FUNCTION "CENTR. 2  ANTERIORE SX" : VOID
TITLE =
VERSION : 0.1

BEGIN
NETWORK
TITLE =LETTURA STATUS WORD DA DRIVE
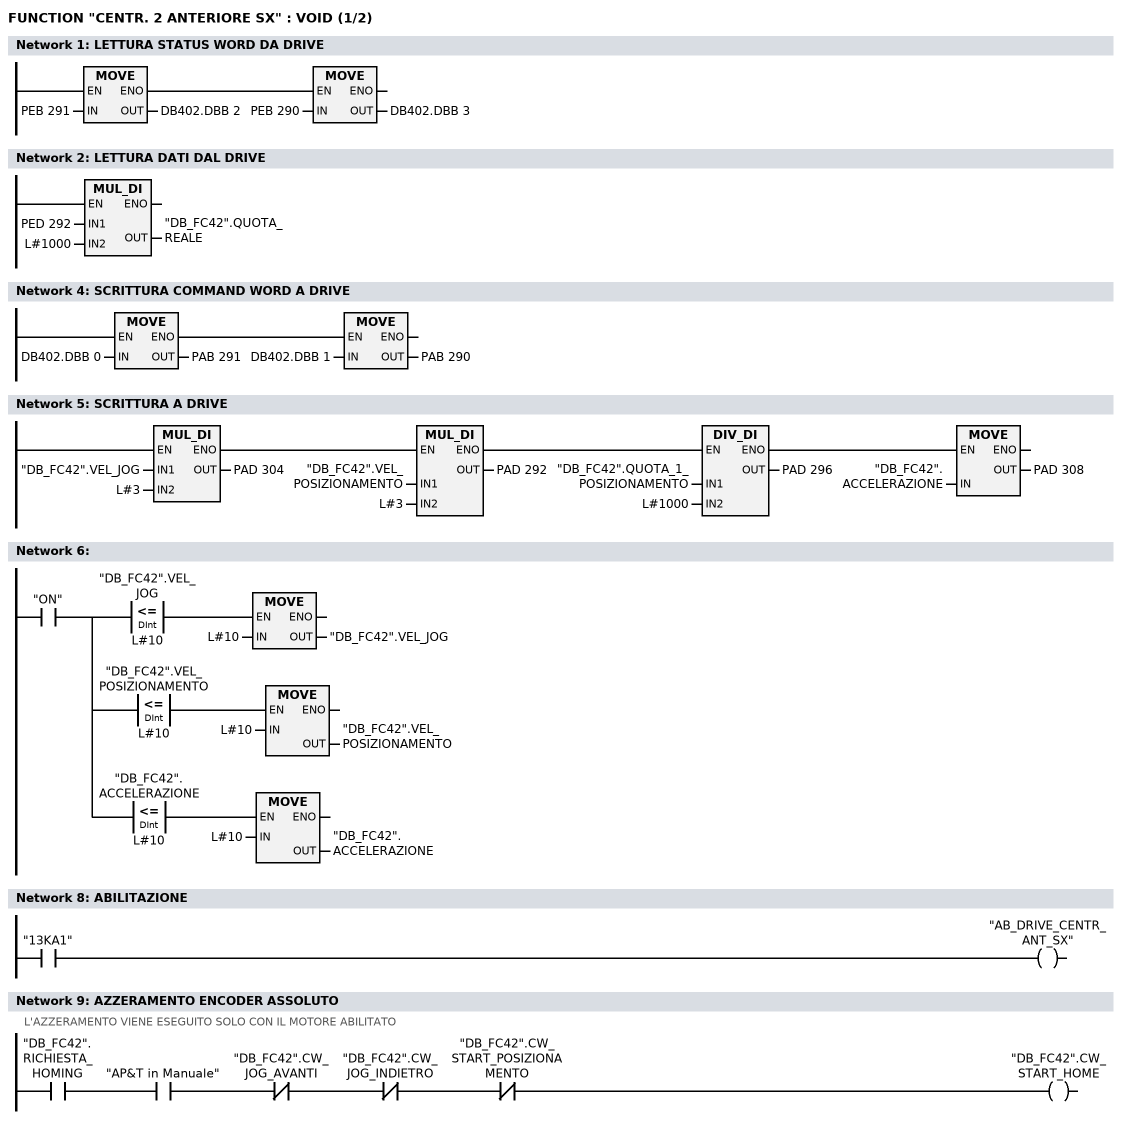
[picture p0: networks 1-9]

      U(    ;
      L     PEB  291;
      T     DB402.DBB    2;
      SET   ;
      SAVE  ;
      CLR   ;
      U     BIE;
      )     ;
      SPBNB _001;
      L     PEB  290;
      T     DB402.DBB    3;
_001: NOP   0;
NETWORK
TITLE =LETTURA DATI DAL DRIVE

      L     PED  292;
      L     L#1000;
      *D    ;
      T     "DB_FC42".QUOTA_REALE;
      NOP   0;
NETWORK
TITLE =

NETWORK
TITLE =SCRITTURA COMMAND WORD A DRIVE

      U(    ;
      L     DB402.DBB    0;
      T     PAB  291;
      SET   ;
      SAVE  ;
      CLR   ;
      U     BIE;
      )     ;
      SPBNB _002;
      L     DB402.DBB    1;
      T     PAB  290;
_002: NOP   0;
NETWORK
TITLE =SCRITTURA A DRIVE

      U(    ;
      U(    ;
      U(    ;
      L     "DB_FC42".VEL_JOG;
      L     L#3;
      *D    ;
      T     PAD  304;
      UN    OV;
      SAVE  ;
      CLR   ;
      U     BIE;
      )     ;
      SPBNB _003;
      L     "DB_FC42".VEL_POSIZIONAMENTO;
      L     L#3;
      *D    ;
      T     PAD  292;
      UN    OV;
      SAVE  ;
      CLR   ;
_003: U     BIE;
      )     ;
      SPBNB _004;
      L     "DB_FC42".QUOTA_1_POSIZIONAMENTO;
      L     L#1000;
      /D    ;
      T     PAD  296;
      UN    OV;
      SAVE  ;
      CLR   ;
_004: U     BIE;
      )     ;
      SPBNB _005;
      L     "DB_FC42".ACCELERAZIONE;
      T     PAD  308;
_005: NOP   0;
NETWORK
TITLE =

      U     "ON";
      =     L      0.0;
      U     L      0.0;
      U(    ;
      L     "DB_FC42".VEL_JOG;
      L     L#10;
      <=D   ;
      )     ;
      SPBNB _006;
      L     L#10;
      T     "DB_FC42".VEL_JOG;
_006: NOP   0;
      U     L      0.0;
      U(    ;
      L     "DB_FC42".VEL_POSIZIONAMENTO;
      L     L#10;
      <=D   ;
      )     ;
      SPBNB _007;
      L     L#10;
      T     "DB_FC42".VEL_POSIZIONAMENTO;
_007: NOP   0;
      U     L      0.0;
      U(    ;
      L     "DB_FC42".ACCELERAZIONE;
      L     L#10;
      <=D   ;
      )     ;
      SPBNB _008;
      L     L#10;
      T     "DB_FC42".ACCELERAZIONE;
_008: NOP   0;
NETWORK
TITLE =

NETWORK
TITLE =ABILITAZIONE

      U     "13KA1";
      =     "AB_DRIVE_CENTR_ANT_SX";
NETWORK
TITLE =AZZERAMENTO ENCODER ASSOLUTO
//L'AZZERAMENTO VIENE ESEGUITO SOLO CON IL MOTORE ABILITATO
      U     "DB_FC42".RICHIESTA_HOMING;
      U     "AP&T in Manuale";
      UN    "DB_FC42".CW_JOG_AVANTI;
      UN    "DB_FC42".CW_JOG_INDIETRO;
      UN    "DB_FC42".CW_START_POSIZIONAMENTO;
      =     "DB_FC42".CW_START_HOME;
NETWORK
TITLE =COMANDI DI JOG
//N.B. VERIFICARE QUOTE EXTRACORSA SOFTWARE
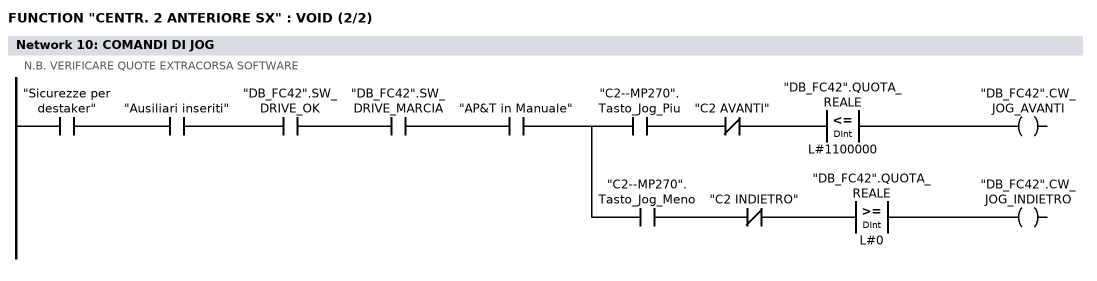
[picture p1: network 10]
      U     "Sicurezze per destaker";
      U     "Ausiliari inseriti";
      U     "DB_FC42".SW_DRIVE_OK;
      U     "DB_FC42".SW_DRIVE_MARCIA;
      U     "AP&T in Manuale";
      =     L      0.0;
      U     L      0.0;
      U     "C2--MP270".Tasto_Jog_Piu;
      UN    "C2 AVANTI";
      U(    ;
      L     "DB_FC42".QUOTA_REALE;
      L     L#1100000;
      <=D   ;
      )     ;
      =     "DB_FC42".CW_JOG_AVANTI;
      U     L      0.0;
      U     "C2--MP270".Tasto_Jog_Meno;
      UN    "C2 INDIETRO";
      U(    ;
      L     "DB_FC42".QUOTA_REALE;
      L     L#0;
      >=D   ;
      )     ;
      =     "DB_FC42".CW_JOG_INDIETRO;
NETWORK
TITLE =Centratore 2: Posizioni

      U     "ON";
      =     L      0.0;
      U     L      0.0;
      U(    ;
      L     "DB_FC42".QUOTA_REALE;
      L     L#100;
      <=D   ;
      )     ;
      U(    ;
      L     "DB_FC42".QUOTA_REALE;
      L     L#-100;
      >=D   ;
      )     ;
      =     "C2: Asse in pos.0";
      U(    ;
      U(    ;
      U     L      0.0;
      SPBNB _009;
      L     "MATRICOLA ATTUALE".C2_Posizione_1;
      L     L#100;
      -D    ;
      T     "CONFRONTI CENTRATORI".C2_Pos_1_Min;
      UN    OV;
      SAVE  ;
      CLR   ;
_009: U     BIE;
      )     ;
      SPBNB _00a;
      L     "MATRICOLA ATTUALE".C2_Posizione_1;
      L     L#200;
      +D    ;
      T     "CONFRONTI CENTRATORI".C2_Pos_1_Max;
      UN    OV;
      SAVE  ;
      CLR   ;
_00a: U     BIE;
      )     ;
      U(    ;
      L     "DB_FC42".QUOTA_REALE;
      L     "CONFRONTI CENTRATORI".C2_Pos_1_Min;
      >=D   ;
      )     ;
      U(    ;
      L     "DB_FC42".QUOTA_REALE;
      L     "CONFRONTI CENTRATORI".C2_Pos_1_Max;
      <=D   ;
      )     ;
      =     "C2: Asse in pos.1";
      U(    ;
      U(    ;
      U     L      0.0;
      SPBNB _00b;
      L     "MATRICOLA ATTUALE".C2_Posizione_2;
      L     L#100;
      -D    ;
      T     "CONFRONTI CENTRATORI".C2_Pos_2_Min;
      UN    OV;
      SAVE  ;
      CLR   ;
_00b: U     BIE;
      )     ;
      SPBNB _00c;
      L     "MATRICOLA ATTUALE".C2_Posizione_2;
      L     L#50000;
      +D    ;
      T     "CONFRONTI CENTRATORI".C2_Pos_2_Max;
      UN    OV;
      SAVE  ;
      CLR   ;
_00c: U     BIE;
      )     ;
      U(    ;
      L     "DB_FC42".QUOTA_REALE;
      L     "CONFRONTI CENTRATORI".C2_Pos_2_Min;
      >=D   ;
      )     ;
      UN    "C2: Asse in pos.3";
      UN    "C2: Asse in pos.4";
      =     "C2: Asse in pos.2";
      U(    ;
      U(    ;
      U     L      0.0;
      SPBNB _00d;
      L     "MATRICOLA ATTUALE".C2_Posizione_3;
      L     L#100;
      -D    ;
      T     "CONFRONTI CENTRATORI".C2_Pos_3_Min;
      UN    OV;
      SAVE  ;
      CLR   ;
_00d: U     BIE;
      )     ;
      SPBNB _00e;
      L     "MATRICOLA ATTUALE".C2_Posizione_3;
      L     L#50000;
      +D    ;
      T     "CONFRONTI CENTRATORI".C2_Pos_3_Max;
      UN    OV;
      SAVE  ;
      CLR   ;
_00e: U     BIE;
      )     ;
      U(    ;
      L     "DB_FC42".QUOTA_REALE;
      L     "CONFRONTI CENTRATORI".C2_Pos_3_Min;
      >=D   ;
      )     ;
      UN    "C2: Asse in pos.4";
      =     "C2: Asse in pos.3";
      U(    ;
      U(    ;
      U     L      0.0;
      SPBNB _00f;
      L     "MATRICOLA ATTUALE".C2_Posizione_4;
      L     L#100;
      -D    ;
      T     "CONFRONTI CENTRATORI".C2_Pos_4_Min;
      UN    OV;
      SAVE  ;
      CLR   ;
_00f: U     BIE;
      )     ;
      SPBNB _010;
      L     "MATRICOLA ATTUALE".C2_Posizione_4;
      L     L#100;
      +D    ;
      T     "CONFRONTI CENTRATORI".C2_Pos_4_Max;
      UN    OV;
      SAVE  ;
      CLR   ;
_010: U     BIE;
      )     ;
      U(    ;
      L     "DB_FC42".QUOTA_REALE;
      L     "CONFRONTI CENTRATORI".C2_Pos_4_Min;
      >=D   ;
      )     ;
      U(    ;
      L     "DB_FC42".QUOTA_REALE;
      L     "CONFRONTI CENTRATORI".C2_Pos_4_Max;
      <=D   ;
      )     ;
      =     "C2: Asse in pos.4";
NETWORK
TITLE =Centratore 2: consenso abilitazione passi
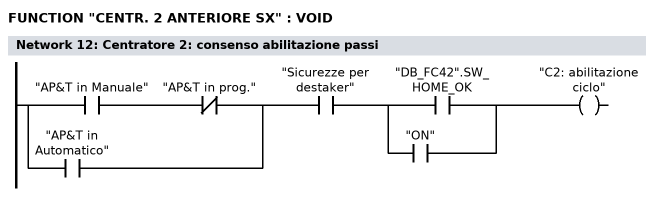
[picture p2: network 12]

      U(    ;
      U     "AP&T in Manuale";
      UN    "AP&T in prog.";
      O     "AP&T in Automatico";
      )     ;
      U     "Sicurezze per destaker";
      U(    ;
      O     "DB_FC42".SW_HOME_OK;
      O     "ON";
      )     ;
      =     "C2: abilitazione ciclo";
NETWORK
TITLE =Centratore 2: comando avvicinamento  (centraggi aperti)

      U(    ;
      U(    ;
      O     "Comando apre centraggi";
      O     "C2--MP270".Tasto_Indietro;
      O     ;
      U     "Apertura centratori";
      U(    ;
      O     "Centratori a riposo";
      O     "Centratori tutti chiusi";
      )     ;
      )     ;
      UN    "C2: Asse in pos.1";
      UN    "C2: comando arrivo";
      UN    "C2: comando a riposo";
      U     "C2: abilitazione ciclo";
      L     S5T#100MS;
      SE    T    183;
      NOP   0;
      NOP   0;
      NOP   0;
      U     T    183;
      )     ;
      S     "C2: comando avvicinam";
      U(    ;
      O     "C2: Asse in pos.1";
      O(    ;
      U(    ;
      O     "Ripristino centratori";
      O     "Comando riposo centraggi";
      O     "C2--MP270".Tasto_Riposo;
      )     ;
      FP    "C2: one shot 1";
      )     ;
      )     ;
      R     "C2: comando avvicinam";
      NOP   0;
NETWORK
TITLE =Centratore 2: comando arrivo (centraggi chiusi)

      U(    ;
      U(    ;
      O     "Comando chiude centraggi";
      O     "C2--MP270".Tasto_Avanti;
      O     ;
      U     "Chiusura centratori";
      U(    ;
      O     "Centratori tutti aperti";
      O     "Centratori a riposo";
      )     ;
      )     ;
      UN    "C2: Asse in pos.4";
      UN    "C2: comando avvicinam";
      UN    "C2: comando a riposo";
      U     "C2: abilitazione ciclo";
      L     S5T#100MS;
      SE    T    184;
      NOP   0;
      NOP   0;
      NOP   0;
      U     T    184;
      )     ;
      S     "C2: comando arrivo";
      U(    ;
      O     "C2: Asse in pos.4";
      O(    ;
      U(    ;
      O     "Ripristino centratori";
      O     "Comando riposo centraggi";
      O     "C2--MP270".Tasto_Riposo;
      )     ;
      FP    "C2: one shot 2";
      )     ;
      )     ;
      R     "C2: comando arrivo";
      NOP   0;
NETWORK
TITLE =Centratore 2: comando automatico centraggi a riposo

      U(    ;
      U(    ;
      O     "Comando riposo centraggi";
      O     "C2--MP270".Tasto_Riposo;
      )     ;
      UN    "C2: Asse in pos.0";
      UN    "C2: comando avvicinam";
      UN    "C2: comando arrivo";
      U     "C2: abilitazione ciclo";
      L     S5T#100MS;
      SE    T    185;
      NOP   0;
      NOP   0;
      NOP   0;
      U     T    185;
      )     ;
      S     "C2: comando a riposo";
      U(    ;
      O     "C2: Asse in pos.0";
      O(    ;
      U     "Ripristino centratori";
      FP    "C2: one shot 3";
      )     ;
      )     ;
      R     "C2: comando a riposo";
      NOP   0;
NETWORK
TITLE =Centratore 2: quote impostate per posizioni

      U     "ON";
      =     L      0.0;
      U(    ;
      U(    ;
      U     L      0.0;
      U     "C2: comando a riposo";
      UN    "C2: Asse in pos.0";
      SPBNB _011;
      L     0;
      T     "DB_FC42".QUOTA_1_POSIZIONAMENTO;
      SET   ;
      SAVE  ;
      CLR   ;
_011: U     BIE;
      )     ;
      SPBNB _012;
      L     L#150;
      T     "DB_FC42".VEL_POSIZIONAMENTO;
      SET   ;
      SAVE  ;
      CLR   ;
_012: U     BIE;
      )     ;
      SPBNB _013;
      L     L#1000;
      T     "DB_FC42".ACCELERAZIONE;
      SET   ;
      SAVE  ;
      CLR   ;
_013: U     BIE;
      =     "C2: Quote pronte pos.0";
      U(    ;
      U(    ;
      U     L      0.0;
      U     "C2: comando avvicinam";
      UN    "C2: Asse in pos.1";
      SPBNB _014;
      L     "MATRICOLA ATTUALE".C2_Posizione_1;
      T     "DB_FC42".QUOTA_1_POSIZIONAMENTO;
      SET   ;
      SAVE  ;
      CLR   ;
_014: U     BIE;
      )     ;
      SPBNB _015;
      L     "MATRICOLA ATTUALE".C2_Velocita_1;
      T     "DB_FC42".VEL_POSIZIONAMENTO;
      SET   ;
      SAVE  ;
      CLR   ;
_015: U     BIE;
      )     ;
      SPBNB _016;
      L     "MATRICOLA ATTUALE".C2_Accell_1;
      T     "DB_FC42".ACCELERAZIONE;
      SET   ;
      SAVE  ;
      CLR   ;
_016: U     BIE;
      =     "C2: Quote pronte pos.1";
      U     L      0.0;
      U     "C2: comando arrivo";
      =     L      0.1;
      U(    ;
      U(    ;
      U     L      0.1;
      UN    "C2: Asse in pos.2";
      SPBNB _017;
      L     "MATRICOLA ATTUALE".C2_Posizione_4;
      T     "DB_FC42".QUOTA_1_POSIZIONAMENTO;
      SET   ;
      SAVE  ;
      CLR   ;
_017: U     BIE;
      )     ;
      SPBNB _018;
      L     "MATRICOLA ATTUALE".C2_Velocita_2;
      T     "DB_FC42".VEL_POSIZIONAMENTO;
      SET   ;
      SAVE  ;
      CLR   ;
_018: U     BIE;
      )     ;
      SPBNB _019;
      L     "MATRICOLA ATTUALE".C2_Accell_2;
      T     "DB_FC42".ACCELERAZIONE;
      SET   ;
      SAVE  ;
      CLR   ;
_019: U     BIE;
      S     "C2: Quote pronte pos.2";
      U     L      0.1;
      U     "C2: Quote pronte pos.2";
      UN    "C2: Reset start pos.2";
      L     S5T#1S;
      SE    "C2: ritardo P2";
      NOP   0;
      NOP   0;
      NOP   0;
      U     "C2: ritardo P2";
      S     "C2: Reset start pos.2";
      R     "C2: Quote pronte pos.2";
      U     L      0.0;
      U     "C2: comando arrivo";
      =     L      0.1;
      U(    ;
      U(    ;
      U(    ;
      U     L      0.1;
      U     "C2: Asse in pos.2";
      UN    "C2: Asse in pos.3";
      SPBNB _01a;
      L     "MATRICOLA ATTUALE".C2_Posizione_4;
      T     "DB_FC42".QUOTA_1_POSIZIONAMENTO;
      SET   ;
      SAVE  ;
      CLR   ;
_01a: U     BIE;
      )     ;
      SPBNB _01b;
      L     "MATRICOLA ATTUALE".C2_Velocita_3;
      T     "DB_FC42".VEL_POSIZIONAMENTO;
      SET   ;
      SAVE  ;
      CLR   ;
_01b: U     BIE;
      )     ;
      SPBNB _01c;
      L     "MATRICOLA ATTUALE".C2_Accell_3;
      T     "DB_FC42".ACCELERAZIONE;
      SET   ;
      SAVE  ;
      CLR   ;
_01c: U     BIE;
      )     ;
      U     "C2: Reset start pos.2";
      S     "C2: Quote pronte pos.3";
      R     "C2: Reset start pos.2";
      U     L      0.1;
      U     "C2: Quote pronte pos.3";
      L     S5T#500MS;
      SE    "C2: ritardo P3";
      NOP   0;
      NOP   0;
      NOP   0;
      U     "C2: ritardo P3";
      S     "C2: Reset start pos.3";
      R     "C2: Quote pronte pos.3";
      U     L      0.0;
      U     "C2: comando arrivo";
      =     L      0.1;
      U(    ;
      U(    ;
      U(    ;
      U     L      0.1;
      U     "C2: Asse in pos.3";
      UN    "C2: Asse in pos.4";
      SPBNB _01d;
      L     "MATRICOLA ATTUALE".C2_Posizione_4;
      T     "DB_FC42".QUOTA_1_POSIZIONAMENTO;
      SET   ;
      SAVE  ;
      CLR   ;
_01d: U     BIE;
      )     ;
      SPBNB _01e;
      L     "MATRICOLA ATTUALE".C2_Velocita_4;
      T     "DB_FC42".VEL_POSIZIONAMENTO;
      SET   ;
      SAVE  ;
      CLR   ;
_01e: U     BIE;
      )     ;
      SPBNB _01f;
      L     "MATRICOLA ATTUALE".C2_Accell_4;
      T     "DB_FC42".ACCELERAZIONE;
      SET   ;
      SAVE  ;
      CLR   ;
_01f: U     BIE;
      )     ;
      U     "C2: Reset start pos.3";
      S     "C2: Quote pronte pos.4";
      R     "C2: Reset start pos.3";
      U     L      0.1;
      U     "C2: Quote pronte pos.4";
      L     S5T#500MS;
      SE    "C2: ritardo P4";
      NOP   0;
      NOP   0;
      NOP   0;
      U     "C2: ritardo P4";
      S     "C2: Reset start pos.4";
      R     "C2: Quote pronte pos.4";
NETWORK
TITLE =Centratore 2: reset impostate
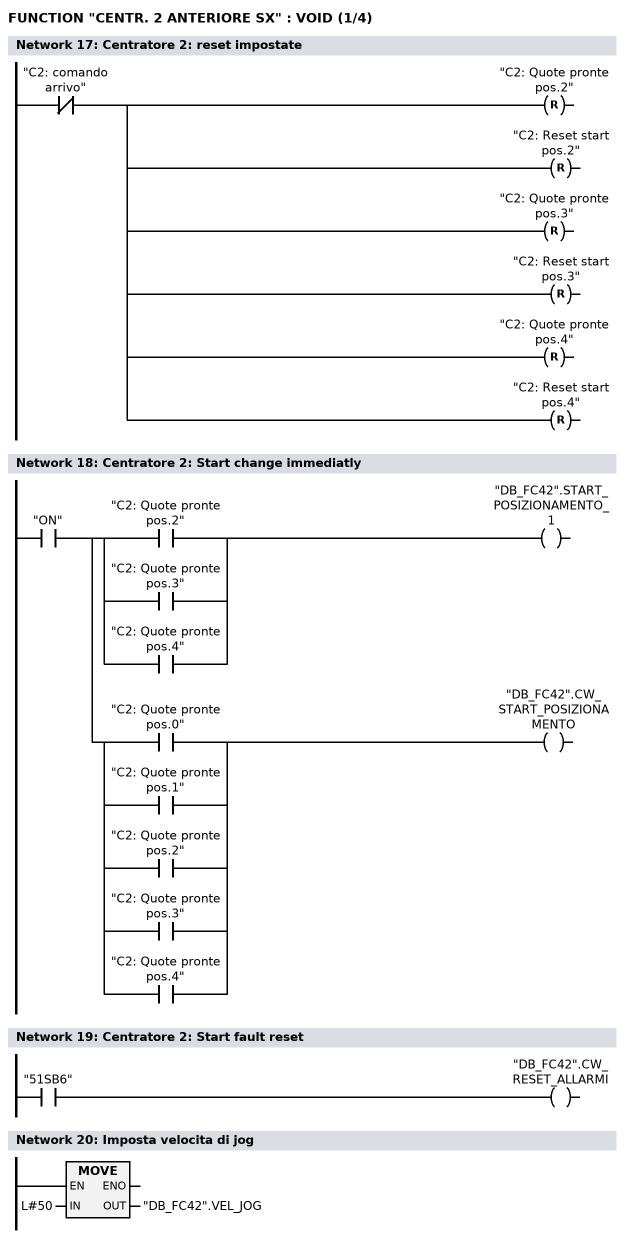
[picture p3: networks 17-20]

      UN    "C2: comando arrivo";
      R     "C2: Quote pronte pos.2";
      R     "C2: Reset start pos.2";
      R     "C2: Quote pronte pos.3";
      R     "C2: Reset start pos.3";
      R     "C2: Quote pronte pos.4";
      R     "C2: Reset start pos.4";
NETWORK
TITLE =Centratore 2: Start change immediatly

      U     "ON";
      =     L      0.0;
      U     L      0.0;
      U(    ;
      O     "C2: Quote pronte pos.2";
      O     "C2: Quote pronte pos.3";
      O     "C2: Quote pronte pos.4";
      )     ;
      =     "DB_FC42".START_POSIZIONAMENTO_1;
      U     L      0.0;
      U(    ;
      O     "C2: Quote pronte pos.0";
      O     "C2: Quote pronte pos.1";
      O     "C2: Quote pronte pos.2";
      O     "C2: Quote pronte pos.3";
      O     "C2: Quote pronte pos.4";
      )     ;
      =     "DB_FC42".CW_START_POSIZIONAMENTO;
NETWORK
TITLE =Centratore 2: Start fault reset

      U     "51SB6";
      =     "DB_FC42".CW_RESET_ALLARMI;
NETWORK
TITLE =Imposta velocita di jog

      L     L#50;
      T     "DB_FC42".VEL_JOG;
      NOP   0;
NETWORK
TITLE =Centratore 1: Drive Enable ok
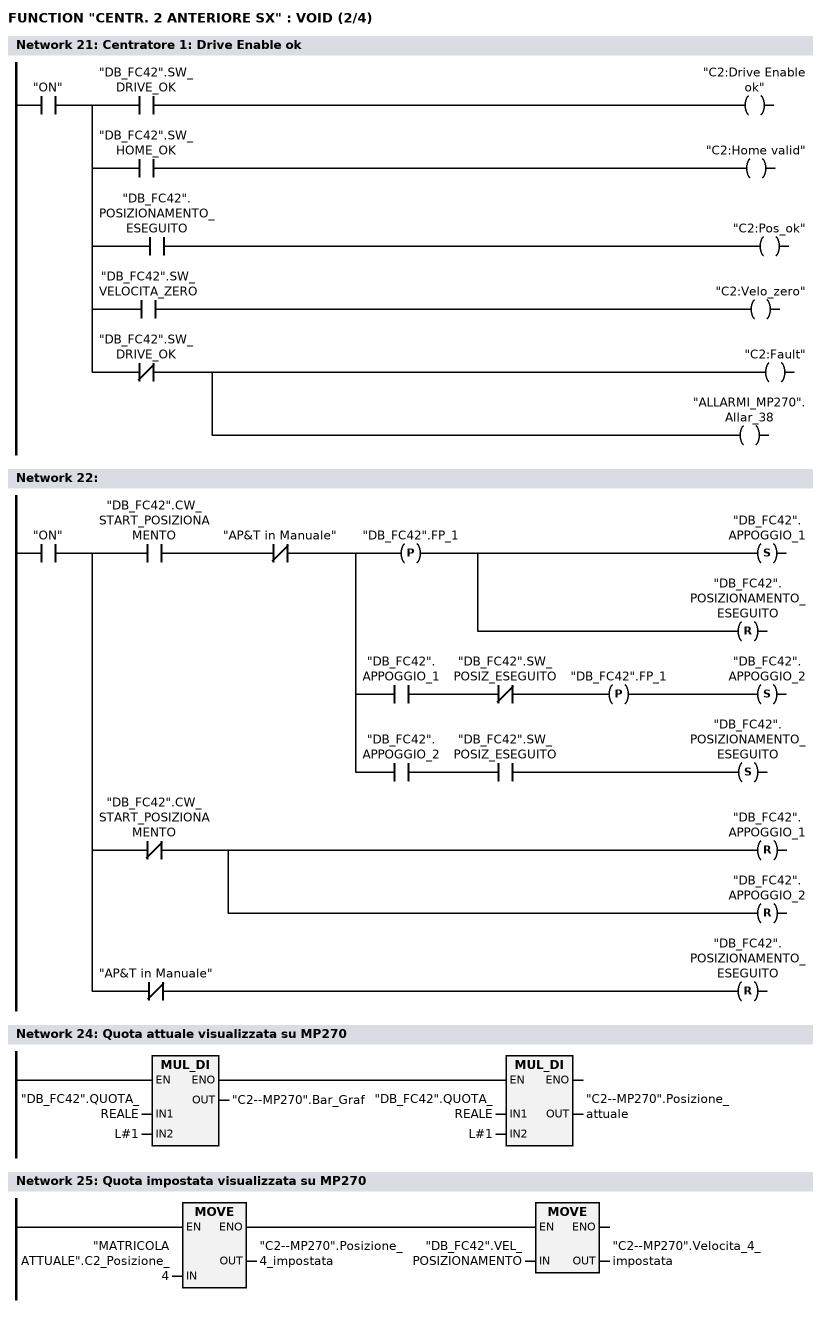
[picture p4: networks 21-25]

      U     "ON";
      =     L      0.0;
      U     L      0.0;
      U     "DB_FC42".SW_DRIVE_OK;
      =     "C2:Drive Enable ok";
      U     L      0.0;
      U     "DB_FC42".SW_HOME_OK;
      =     "C2:Home valid";
      U     L      0.0;
      U     "DB_FC42".POSIZIONAMENTO_ESEGUITO;
      =     "C2:Pos_ok";
      U     L      0.0;
      U     "DB_FC42".SW_VELOCITA_ZERO;
      =     "C2:Velo_zero";
      U     L      0.0;
      UN    "DB_FC42".SW_DRIVE_OK;
      =     "C2:Fault";
      =     "ALLARMI_MP270".Allar_38;
NETWORK
TITLE =

      U     "ON";
      =     L      0.0;
      U     L      0.0;
      U     "DB_FC42".CW_START_POSIZIONAMENTO;
      UN    "AP&T in Manuale";
      =     L      0.1;
      U     L      0.1;
      FP    "DB_FC42".FP_1;
      S     "DB_FC42".APPOGGIO_1;
      R     "DB_FC42".POSIZIONAMENTO_ESEGUITO;
      U     L      0.1;
      U     "DB_FC42".APPOGGIO_1;
      UN    "DB_FC42".SW_POSIZ_ESEGUITO;
      FP    "DB_FC42".FP_1;
      S     "DB_FC42".APPOGGIO_2;
      U     L      0.1;
      U     "DB_FC42".APPOGGIO_2;
      U     "DB_FC42".SW_POSIZ_ESEGUITO;
      S     "DB_FC42".POSIZIONAMENTO_ESEGUITO;
      U     L      0.0;
      UN    "DB_FC42".CW_START_POSIZIONAMENTO;
      R     "DB_FC42".APPOGGIO_1;
      R     "DB_FC42".APPOGGIO_2;
      U     L      0.0;
      UN    "AP&T in Manuale";
      R     "DB_FC42".POSIZIONAMENTO_ESEGUITO;
NETWORK
TITLE =

NETWORK
TITLE =Quota attuale visualizzata su MP270

      U(    ;
      L     "DB_FC42".QUOTA_REALE;
      L     L#1;
      *D    ;
      T     "C2--MP270".Bar_Graf;
      UN    OV;
      SAVE  ;
      CLR   ;
      U     BIE;
      )     ;
      SPBNB _020;
      L     "DB_FC42".QUOTA_REALE;
      L     L#1;
      *D    ;
      T     "C2--MP270".Posizione_attuale;
_020: NOP   0;
NETWORK
TITLE =Quota impostata visualizzata su MP270

      U(    ;
      L     "MATRICOLA ATTUALE".C2_Posizione_4;
      T     "C2--MP270".Posizione_4_impostata;
      SET   ;
      SAVE  ;
      CLR   ;
      U     BIE;
      )     ;
      SPBNB _021;
      L     "DB_FC42".VEL_POSIZIONAMENTO;
      T     "C2--MP270".Velocita_4_impostata;
_021: NOP   0;
NETWORK
TITLE =Visualizza FC su MP270
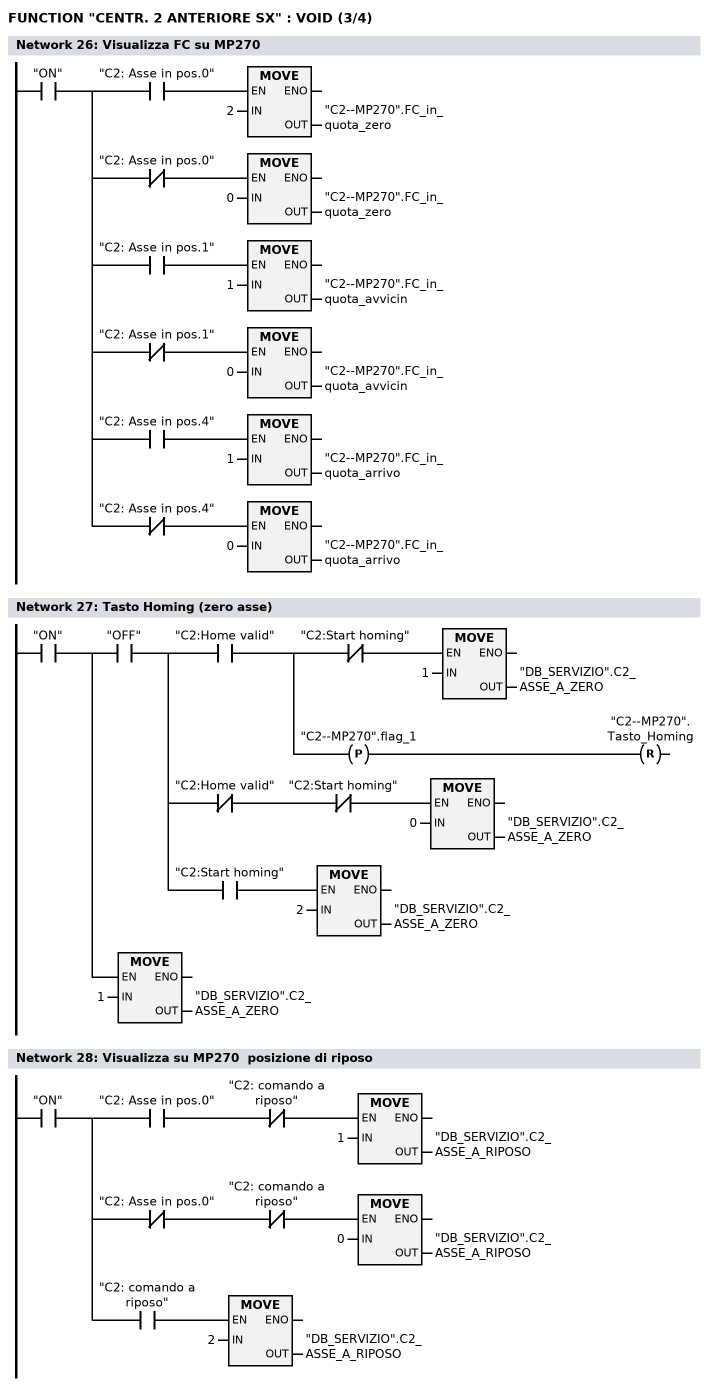
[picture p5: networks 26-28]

      U     "ON";
      =     L      0.0;
      U     L      0.0;
      U     "C2: Asse in pos.0";
      SPBNB _022;
      L     2;
      T     "C2--MP270".FC_in_quota_zero;
_022: NOP   0;
      U     L      0.0;
      UN    "C2: Asse in pos.0";
      SPBNB _023;
      L     0;
      T     "C2--MP270".FC_in_quota_zero;
_023: NOP   0;
      U     L      0.0;
      U     "C2: Asse in pos.1";
      SPBNB _024;
      L     1;
      T     "C2--MP270".FC_in_quota_avvicin;
_024: NOP   0;
      U     L      0.0;
      UN    "C2: Asse in pos.1";
      SPBNB _025;
      L     0;
      T     "C2--MP270".FC_in_quota_avvicin;
_025: NOP   0;
      U     L      0.0;
      U     "C2: Asse in pos.4";
      SPBNB _026;
      L     1;
      T     "C2--MP270".FC_in_quota_arrivo;
_026: NOP   0;
      U     L      0.0;
      UN    "C2: Asse in pos.4";
      SPBNB _027;
      L     0;
      T     "C2--MP270".FC_in_quota_arrivo;
_027: NOP   0;
NETWORK
TITLE =Tasto Homing (zero asse)

      U     "ON";
      =     L      0.0;
      U     L      0.0;
      U     "OFF";
      =     L      0.1;
      U     L      0.1;
      U     "C2:Home valid";
      =     L      0.2;
      U     L      0.2;
      UN    "C2:Start homing";
      SPBNB _028;
      L     1;
      T     "DB_SERVIZIO".C2_ASSE_A_ZERO;
_028: NOP   0;
      U     L      0.2;
      FP    "C2--MP270".flag_1;
      R     "C2--MP270".Tasto_Homing;
      U     L      0.1;
      UN    "C2:Home valid";
      UN    "C2:Start homing";
      SPBNB _029;
      L     0;
      T     "DB_SERVIZIO".C2_ASSE_A_ZERO;
_029: NOP   0;
      U     L      0.1;
      U     "C2:Start homing";
      SPBNB _02a;
      L     2;
      T     "DB_SERVIZIO".C2_ASSE_A_ZERO;
_02a: NOP   0;
      U     L      0.0;
      SPBNB _02b;
      L     1;
      T     "DB_SERVIZIO".C2_ASSE_A_ZERO;
_02b: NOP   0;
NETWORK
TITLE =Visualizza su MP270  posizione di riposo

      U     "ON";
      =     L      0.0;
      U     L      0.0;
      U     "C2: Asse in pos.0";
      UN    "C2: comando a riposo";
      SPBNB _02c;
      L     1;
      T     "DB_SERVIZIO".C2_ASSE_A_RIPOSO;
_02c: NOP   0;
      U     L      0.0;
      UN    "C2: Asse in pos.0";
      UN    "C2: comando a riposo";
      SPBNB _02d;
      L     0;
      T     "DB_SERVIZIO".C2_ASSE_A_RIPOSO;
_02d: NOP   0;
      U     L      0.0;
      U     "C2: comando a riposo";
      SPBNB _02e;
      L     2;
      T     "DB_SERVIZIO".C2_ASSE_A_RIPOSO;
_02e: NOP   0;
NETWORK
TITLE =Visualizza su MP270  posizione di avvicinamento
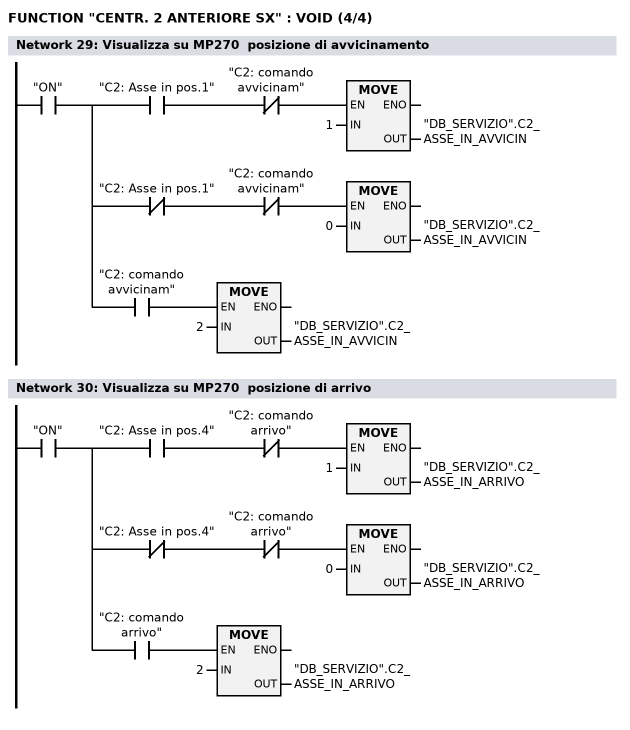
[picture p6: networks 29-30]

      U     "ON";
      =     L      0.0;
      U     L      0.0;
      U     "C2: Asse in pos.1";
      UN    "C2: comando avvicinam";
      SPBNB _02f;
      L     1;
      T     "DB_SERVIZIO".C2_ASSE_IN_AVVICIN;
_02f: NOP   0;
      U     L      0.0;
      UN    "C2: Asse in pos.1";
      UN    "C2: comando avvicinam";
      SPBNB _030;
      L     0;
      T     "DB_SERVIZIO".C2_ASSE_IN_AVVICIN;
_030: NOP   0;
      U     L      0.0;
      U     "C2: comando avvicinam";
      SPBNB _031;
      L     2;
      T     "DB_SERVIZIO".C2_ASSE_IN_AVVICIN;
_031: NOP   0;
NETWORK
TITLE =Visualizza su MP270  posizione di arrivo

      U     "ON";
      =     L      0.0;
      U     L      0.0;
      U     "C2: Asse in pos.4";
      UN    "C2: comando arrivo";
      SPBNB _032;
      L     1;
      T     "DB_SERVIZIO".C2_ASSE_IN_ARRIVO;
_032: NOP   0;
      U     L      0.0;
      UN    "C2: Asse in pos.4";
      UN    "C2: comando arrivo";
      SPBNB _033;
      L     0;
      T     "DB_SERVIZIO".C2_ASSE_IN_ARRIVO;
_033: NOP   0;
      U     L      0.0;
      U     "C2: comando arrivo";
      SPBNB _034;
      L     2;
      T     "DB_SERVIZIO".C2_ASSE_IN_ARRIVO;
_034: NOP   0;
END_FUNCTION

